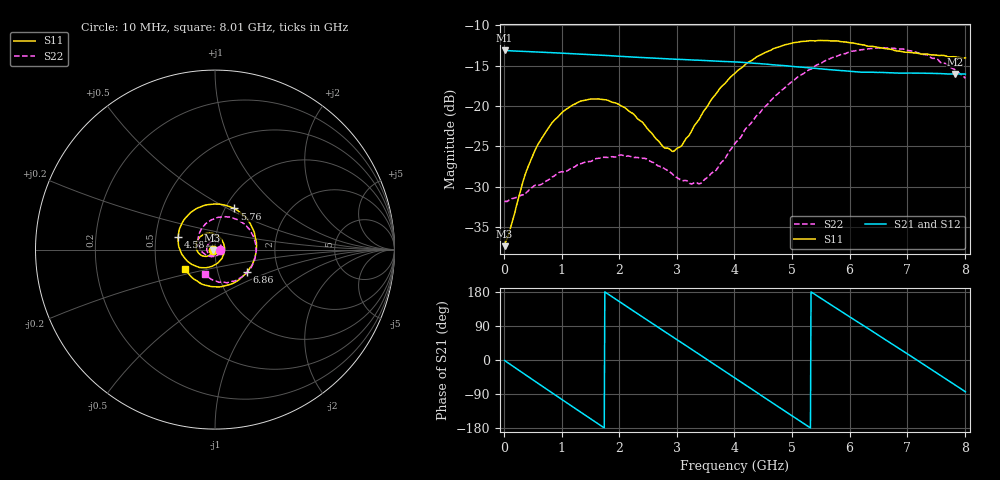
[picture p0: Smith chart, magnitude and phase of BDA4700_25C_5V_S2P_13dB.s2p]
!Agilent Technologies,E5071B,MY42404982,A.09.10
!Date: Mon Oct 20 13:32:39 2025
!Data & Calibration Information:
!Freq	S11:SOLT2(ON)	S21:SOLT2(ON)	S12:SOLT2(ON)	S22:SOLT2(ON)
# Hz S RI R 50
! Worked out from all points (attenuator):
!   801 points, 10 MHz to 8.01 GHz, reference 50 ohm
!   highest |S21| = -13.11 dB at 10 MHz (marker M1); lowest = -16.1 dB at 7.83 GHz (marker M2)
!   lowest |S11| = -37.4 dB at 10 MHz (marker M3), VSWR 1.03, Z = 48.7 - j0.149 ohm
!   |S11| at or under -10 dB: start of sweep to end of sweep
!   |S22| runs from -31.8 to -12.8 dB; largest |S21 - S12| = 0.0016
!   S11 on the Smith chart (normalised r, x): 10 MHz: 0.97, -0.00; 4.58 GHz: 0.65, +0.10; 5.76 GHz: 1.10, +0.54; 6.86 GHz: 1.38, -0.36; 8.01 GHz: 0.70, -0.15
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1e7  -0.0135 -0.00153  0.221 -0.00475  0.221 -0.00502  0.0257 -0.000998
3.6e8  -0.0253 -0.027  0.1719 -0.1332  0.1718 -0.1334  0.0214 -0.0189
5.8e8  -0.0433 -0.0371  0.1063 -0.1879  0.1062 -0.188  0.0127 -0.0299
8.8e8  -0.0754 -0.0325  -0.00512 -0.2133  -0.00514 -0.2134  -0.0103 -0.0356
1.35e9  -0.1061 0.018  -0.1591 -0.1359  -0.1592 -0.1359  -0.042 -0.0135
1.94e9  -0.0569 0.0875  -0.192 0.0683  -0.1921 0.0684  -0.0316 0.0366
2.33e9  0.00609 0.0824  -0.1031 0.1714  -0.1032 0.1714  0.00108 0.0479
2.68e9  0.0466 0.0389  0.014 0.1967  0.014 0.1967  0.028 0.0319
2.96e9  0.051 -0.0135  0.1035 0.1649  0.1036 0.1648  0.0357 0.00927
3.4e9  -0.000646 -0.084  0.1863 0.0458  0.1865 0.0457  0.0177 -0.0279
3.69e9  -0.0651 -0.1008  0.1829 -0.0499  0.1829 -0.0505  -0.0113 -0.0387
4.01e9  -0.1415 -0.0738  0.1265 -0.1383  0.1265 -0.1381  -0.0494 -0.0311
4.58e9  -0.2051 0.0726  -0.0472 -0.1749  -0.0471 -0.1751  -0.093 0.0441
4.92e9  -0.1656 0.175  -0.1341 -0.1156  -0.1339 -0.1162  -0.0791 0.1086
5.35e9  -0.0402 0.2502  -0.1714 0.00636  -0.1715 0.00588  -0.00478 0.1705
5.76e9  0.1071 0.2293  -0.1227 0.1127  -0.1225 0.1128  0.1002 0.1758
6.23e9  0.2175 0.0987  -0.00514 0.1616  -0.00365 0.1617  0.2024 0.094
6.68e9  0.2151 -0.0669  0.108 0.1187  0.1083 0.1187  0.2252 -0.0327
6.86e9  0.1796 -0.1242  0.1382 0.0803  0.1385 0.0796  0.209 -0.0837
7.34e9  0.0293 -0.2074  0.1522 -0.047  0.1523 -0.0472  0.1117 -0.1744
7.83e9  -0.13 -0.1541  0.065 -0.1435  0.0648 -0.1438  -0.0189 -0.1664
8.01e9  -0.1681 -0.1058  0.0166 -0.1567  0.017 -0.1568  -0.0564 -0.1373
